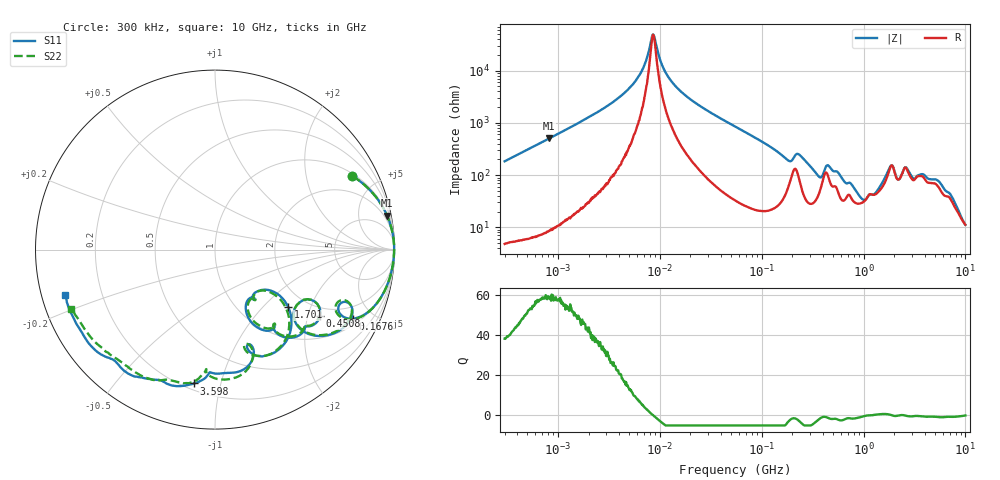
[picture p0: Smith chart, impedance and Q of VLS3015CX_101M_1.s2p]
! S-Parameter Data Generated by TDK Corporation
! Copyright(C) 2019 TDK Corporation.
! All Rights Reserved.
! TDK P/N: VLS3015CX-101M-1 (Inductor)
! Property: L=100uH at 1MHz
! Size(LxWxT): 3x3x1.5mm
! Model Type: s2p (Touchstone File Format Version 1.0)
! Frequency: DC=Yes Start=0.3MHz Stop=10000MHz 802points Log-sweep
! Model Generated on Sep. 23, 2019
! Port Assignments:
!  1 ---@@@--- 2
! Applicable Conditions:
!  Temperature = 25 degC
!  DC Bias Current = 0 A
!  Small Signal Operation
! Terms and conditions regarding TDK Simulation Models
! (1)This simulation model is being provided solely for informational purposes. Please refer to the specifications of the products in terms of detailed characteristics of such products.
! (2)In no event shall TDK Corporation of any of its subsidiaries be liable for any loss or damage arising, directly or indirectly,
!  From any information contained in this simulation model, including, but not limited to loss or damages arising from any inaccuracies, omissions or errors in connection with such information.
! (3)Any and all copyrights on this simulation model are owned by TDK Corporation.
!  Duplication or redistribution of this simulation model without prior written permission from TDK Corporation is prohibited.
! (4)This simulation model is subject to any modification or change without any prior notice.
! (5)Neither TDK Corporation nor any of its subsidiaries shall make any warranty, express or implied,
!  Including but not limited to the correctness, implied warranties of merchantability and fitness for a particular purpose with respect to this simulation models.
! (6)The use of this simulation model shall be deemed to have consented to the terms and conditions hereof.
# Hz S MA R 50
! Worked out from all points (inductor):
!   801 points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, 300 kHz to 10 GHz, reference 50 ohm
!   read as one part in series: L = 97.3 uH near 318.3 kHz
!   highest Q = 58.5 at 820.8 kHz (marker M1), where L = 97.5 uH
!   self-resonance near 8.603 MHz
!   S11 on the Smith chart (normalised r, x): 300 kHz: 1.10, +3.68; 167.6 MHz: 1.29, -3.83; 450.8 MHz: 1.68, -2.40; 1.701 GHz: 1.61, -1.42; 3.598 GHz: 0.24, -0.83; 10 GHz: 0.07, -0.15
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300000  0.8687 28.1  0.4727 -60.4  0.4728 -60.4  0.8686 28.1
820758  0.9774 11.2  0.1944 -77.8  0.1944 -77.8  0.9772 11.2
1713600  0.9938 5.2  0.09229 -83.5  0.09218 -83.5  0.9937 5.2
5292453  0.9982 1.0  0.01944 -84.2  0.01939 -84.0  0.9981 1.0
6899350  0.9982 0.3  0.008774 -77.5  0.008732 -77.7  0.9981 0.3
8484346  0.998 -0.2  0.002059 -17.5  0.002101 -18.3  0.998 -0.2
9671944  0.9979 -0.5  0.004736 64.0  0.004752 64.0  0.998 -0.5
1.49005e7  0.9975 -1.6  0.02155 82.3  0.02156 82.3  0.9975 -1.7
5.477226e7  0.9889 -8.1  0.1155 79.7  0.1156 79.7  0.9888 -8.2
1.6757e8  0.8607 -26.5  0.3849 53.2  0.3849 53.2  0.8558 -27.1
2.257919e8  0.8319 -23.2  0.3172 42.8  0.3172 42.8  0.8222 -22.6
3.126428e8  0.7529 -39.7  0.5256 39.0  0.5256 39.0  0.7517 -39.4
3.730642e8  0.5743 -40.3  0.5787 19.6  0.5787 19.6  0.5742 -40.1
4.508285e8  0.6926 -32.3  0.4232 22.3  0.4232 22.3  0.69 -32.4
6.076905e8  0.6308 -51.0  0.5954 20.3  0.5955 20.3  0.6269 -50.5
9.67469e8  0.3783 -62.9  0.7219 -7.9  0.7218 -7.9  0.3869 -61.6
1.371335e9  0.3309 -44.9  0.6523 -33.8  0.6522 -33.7  0.3367 -43.2
1.701119e9  0.5198 -38.2  0.4734 -53.0  0.4736 -53.0  0.5247 -40.2
1.767019e9  0.5753 -42.3  0.4174 -53.7  0.4176 -53.7  0.5753 -44.0
3.598403e9  0.7548 -99.0  0.308 -55.1  0.3081 -55.2  0.7047 -96.1
5.849356e9  0.8435 -125.1  0.2671 -59.3  0.2674 -59.4  0.8151 -123.0
1e10  0.8709 -163.0  0.2289 -88.4  0.2291 -88.3  0.8691 -157.5
